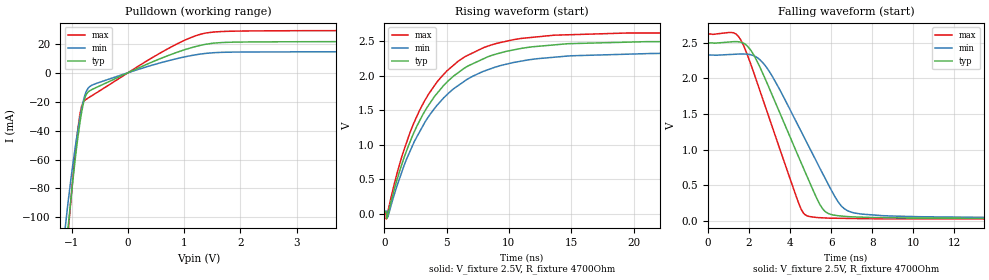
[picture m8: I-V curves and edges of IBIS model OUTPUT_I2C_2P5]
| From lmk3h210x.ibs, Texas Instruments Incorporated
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[Model]   OUTPUT_I2C_2P5
Model_type   Open_drain
Polarity   Non-Inverting
Vmeas = 1.25
Vref = 2.5
Cref = 10pF
Rref = 4700
|   typ   min   max
C_comp   0.7pF   0.5pF   0.9pF
[Voltage Range]   2.5   2.375   2.625
[Temperature Range]   45   125   -40
[Pullup Reference]   2.5   2.375   2.625
[Pulldown Reference]   0   0   0
[Power Clamp Reference]   2.5   2.375   2.625
[GND Clamp Reference]   0   0   0
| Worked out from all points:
|   slope of the pulldown table from 0 to 0.375 V, typ, clamps not added: 57.3 ohm
|   falling waveform, V_fixture 2.5V, R_fixture 4700Ohm: 20-80 % time 2.21ns typ, 2.45ns min, 1.85ns max; typ from 2.5 V to 0.029 V
|   rising waveform, V_fixture 2.5V, R_fixture 4700Ohm: 20-80 % time 4.57ns typ, 4.85ns min, 4.29ns max; typ from 0.029 V to 2.5 V
[Pulldown]
|   Voltage   I(typ)   I(min)   I(max)
-3.3V     -1.111A    -994.6mA   -1.235A
-1.181V   -155mA     -130.2mA   -166mA
-1.063V   -106.3mA   -88.93mA   -110.1mA
-1.013V   -87.04mA   -73.2mA    -87.67mA
-914.1mV  -52.02mA   -45.46mA   -46.91mA
-854.7mV  -34.77mA   -31.34mA   -28.74mA
-795.3mV  -21.66mA   -19.82mA   -20.37mA
-735.9mV  -14.64mA   -12.47mA   -18.18mA
16.5mV    299uA      212.7uA    413.8uA
1.214V    18.26mA    12.49mA    25.72mA
1.828V    21.11mA    14.25mA    28.71mA
6.6V      22.24mA    14.99mA    30.18mA
[Ramp]
R_load = 4700
|   typ   min   max
dV/dt_r   1.48257/4.57046e-09   1.375/4.82427e-09   1.56174/4.27227e-09
dV/dt_f   1.48257/2.2077e-09   1.37491/2.44615e-09   1.56174/1.85398e-09
[Falling Waveform]
V_fixture = 2.5V
V_fixture_min = 2.375V
V_fixture_max = 2.625V
R_fixture = 4700Ohm
C_fixture = 0F
|   Time   V(typ)   V(min)   V(max)
0s        2.5V       2.33V      2.625V
1.223ns   2.517V     2.339V     2.644V
1.587ns   2.512V     2.345V     2.546V
2.147ns   2.369V     2.328V     2.148V
2.841ns   1.958V     2.16V      1.563V
4.64ns    746.2mV    1.198V     111.1mV
5.704ns   129.7mV    597.6mV    37.71mV
6.495ns   64.43mV    207.2mV    32.23mV
7.545ns   48.07mV    90.89mV    27.6mV
1.25us    29.05mV    38.66mV    22.09mV
[Rising Waveform]
V_fixture = 2.5V
V_fixture_min = 2.375V
V_fixture_max = 2.625V
R_fixture = 4700Ohm
C_fixture = 0F
|   Time   V(typ)   V(min)   V(max)
0s        29.05mV    38.66mV    22.09mV
169.3ps   17.3mV     38.13mV    -76.33mV
286.5ps   -18.11mV   -47.56mV   23.52mV
1.471ns   748.9mV    637.3mV    864.5mV
2.785ns   1.328V     1.17V      1.479V
4.176ns   1.73V      1.558V     1.895V
5.904ns   2.04V      1.853V     2.205V
11.06ns   2.397V     2.212V     2.54V
19.47ns   2.484V     2.31V      2.617V
1.25us    2.5V       2.33V      2.625V
